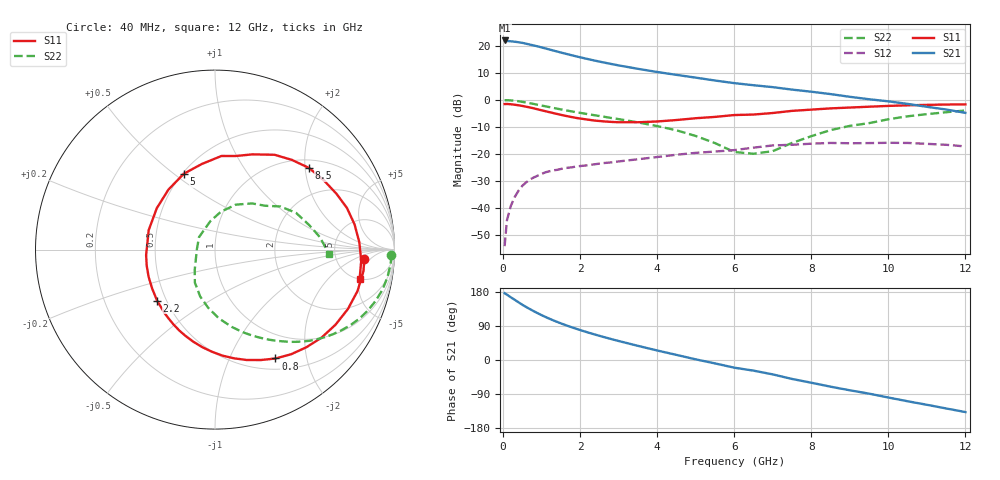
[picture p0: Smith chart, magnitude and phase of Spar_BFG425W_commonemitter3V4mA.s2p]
! Filename: 34bfg425.001
! BFG425W Field C1
! V1=8.204E-001V,V2=3.000E+000V, I1=4.819E-005A, I2=4.000E-003A
# GHz  S  MA  R 50
!  S11  S21  S12  S22
!Freq(GHz)  Mag  Ang  Mag  Ang  Mag  Ang  Mag  Ang
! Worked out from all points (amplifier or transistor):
!   44 points, 40 MHz to 12 GHz, reference 50 ohm
!   highest |S21| = 21.9 dB at 40 MHz (marker M1)
!   |S21| within 3 dB of that: start of sweep to 1.115 GHz
!   unconditionally stable (mu >= 1): 2.635 GHz to end of sweep
!   at 700 MHz: K = 0.29, MSG = 24.9 dB, |S12| = -29.4 dB
!   at 2.4 GHz: K = 0.93, MSG = 19.1 dB, |S12| = -23.7 dB
!   at 12 GHz: K = 1.55, MAG = 1.8 dB, |S12| = -17.2 dB
!   S11 on the Smith chart (normalised r, x): 40 MHz: 10, -3; 800 MHz: 0.64, -1.50; 2.2 GHz: 0.45, -0.31; 5 GHz: 0.51, +0.54; 8.5 GHz: 1.20, +2.10; 12 GHz: 5.05, -5.07
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0.04  0.833 -3.6  12.4 176.3  0.002 70.3  0.983 -1.8
0.1  0.836 -8.2  12.11 172.5  0.006 82.3  0.982 -4.6
0.3  0.811 -24.2  11.76 159.1  0.016 74.3  0.959 -13.6
0.5  0.77 -39.6  11.21 145.8  0.026 66.0  0.916 -21.9
0.6  0.745 -47.0  10.8 139.8  0.03 61.9  0.891 -25.6
0.8  0.694 -60.9  10.02 128.6  0.037 55.0  0.836 -32.5
1.1  0.615 -80.1  8.837 113.6  0.046 46.5  0.757 -41.2
1.3  0.569 -91.8  8.099 104.8  0.05 42.0  0.709 -46.3
1.5  0.528 -103.0  7.438 96.7  0.053 38.3  0.665 -50.6
1.8  0.477 -118.9  6.569 85.7  0.057 34.0  0.607 -56.6
2.2  0.43 -138.6  5.629 72.8  0.062 29.5  0.543 -63.9
2.6  0.4 -157.5  4.89 61.0  0.068 26.1  0.489 -70.9
3  0.385 -175.4  4.302 50.1  0.073 23.0  0.44 -77.9
3.5  0.385 163.6  3.721 37.4  0.08 18.9  0.383 -86.9
4.5  0.423 127.9  2.879 13.5  0.097 9.3  0.274 -107.5
5  0.457 112.4  2.559 1.7  0.105 2.5  0.215 -121.5
6  0.523 86.0  2.027 -20.3  0.118 -10.5  0.109 -163.2
6.5  0.534 77.6  1.854 -28.1  0.131 -11.1  0.101 178.8
7.5  0.624 57.9  1.54 -50.0  0.148 -29.8  0.16 99.5
8.5  0.694 40.9  1.273 -70.4  0.16 -46.5  0.276 65.2
10.5  0.79 10.3  0.84 -108.9  0.16 -81.6  0.496 24.3
12  0.822 -11.4  0.574 -137.4  0.138 -112.7  0.635 -2.2
